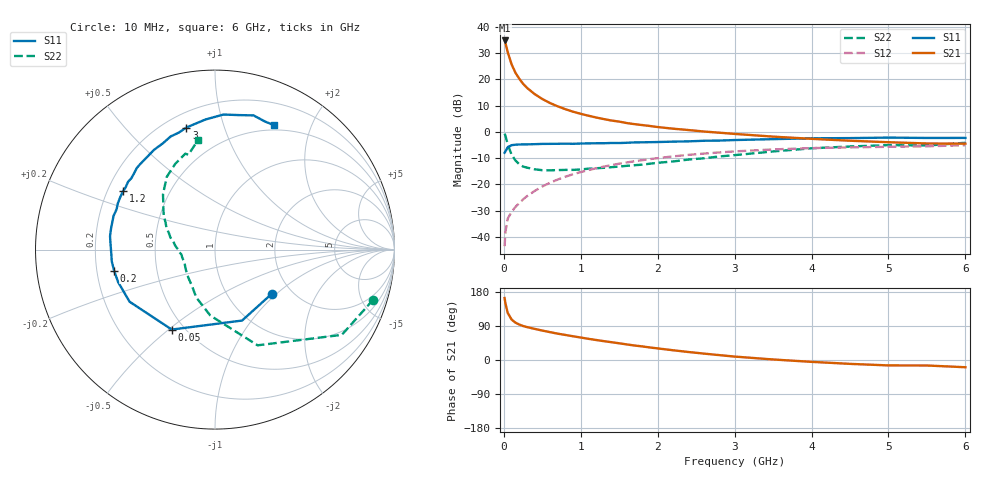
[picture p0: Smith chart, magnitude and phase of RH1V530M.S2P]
! SIEMENS Small Signal Semiconductors
! BFR106
! Si NPN RF Bipolar Junction Transistor in SOT23
! VCE = 1.5 V  IC = 30 mA
! Common Emitter S-Parameters:  August  1996
# GHz  S  MA  R  50
!  f  S11  S21  S12  S22
! GHz  MAG  ANG  MAG  ANG  MAG  ANG  MAG  ANG
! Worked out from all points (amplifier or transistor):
!   36 points, 10 MHz to 6 GHz, reference 50 ohm
!   highest |S21| = 34.9 dB at 10 MHz (marker M1)
!   |S21| within 3 dB of that: start of sweep to 37.96 MHz
!   unconditionally stable (mu >= 1): 283.2 MHz to 2.885 GHz; 4.796 GHz to end of sweep
!   at 250 MHz: K = 0.97, MSG = 22.1 dB, |S12| = -25.7 dB
!   at 1.4 GHz: K = 1.07, MAG = 6.8 dB, |S12| = -12.7 dB
!   at 6 GHz: K = 1.02, MAG = -0.5 dB, |S12| = -5.1 dB
!   S11 on the Smith chart (normalised r, x): 10 MHz: 1.59, -0.93; 50 MHz: 0.43, -0.51; 200 MHz: 0.27, -0.09; 1.2 GHz: 0.26, +0.27; 3 GHz: 0.28, +0.75; 6 GHz: 0.44, +1.49
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0.01  0.4008 -38.0  55.5 163.6  0.0066 79.9  0.9245 -17.6
0.02  0.4231 -69.1  50.02 150.2  0.0122 66.7  0.8514 -33.9
0.05  0.5064 -118.4  33.42 124.5  0.022 54.9  0.5838 -66.0
0.1  0.5575 -148.6  19.59 107.0  0.0298 53.4  0.3681 -94.1
0.15  0.5694 -161.5  13.5 98.6  0.0369 56.5  0.2862 -111.4
0.2  0.5744 -168.3  10.33 93.6  0.0437 60.1  0.241 -121.9
0.25  0.5788 -173.4  8.283 89.7  0.0516 61.8  0.2181 -132.1
0.3  0.5781 -177.1  6.945 86.9  0.0592 64.1  0.2081 -138.3
0.4  0.5829 176.9  5.264 82.1  0.0745 66.1  0.1933 -148.6
0.5  0.5896 172.7  4.235 77.7  0.091 66.6  0.1858 -155.6
0.6  0.591 168.5  3.552 73.5  0.1069 66.6  0.1848 -160.1
0.7  0.5927 164.4  3.072 69.5  0.1232 66.0  0.1866 -164.1
0.9  0.5924 157.8  2.427 62.6  0.1556 64.0  0.1883 -171.1
1.1  0.6034 151.0  2.032 55.9  0.187 61.5  0.1984 -175.6
1.2  0.607 147.7  1.881 52.8  0.2022 60.1  0.2024 -178.2
1.6  0.6199 136.6  1.472 41.0  0.2615 53.8  0.2253 173.3
2.2  0.6516 121.3  1.151 25.7  0.3408 43.8  0.2724 160.4
3  0.6987 103.2  0.915 9.0  0.4243 30.5  0.3598 143.0
3.5  0.7268 94.2  0.812 1.4  0.4629 22.9  0.4231 133.2
4.5  0.7612 79.9  0.678 -10.2  0.5061 8.6  0.5266 114.9
5.5  0.7659 68.6  0.601 -14.5  0.5311 -0.1  0.5489 105.7
6  0.7675 64.7  0.596 -19.1  0.556 -6.8  0.6198 98.6
